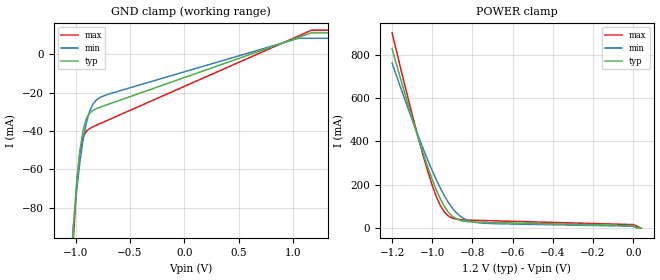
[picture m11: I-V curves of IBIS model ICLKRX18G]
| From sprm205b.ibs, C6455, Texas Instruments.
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|   Model ICLKRX18G
[Model]   ICLKRX18G
Model_type   Input
Polarity   Non-Inverting
C_comp   2.6600pF   1.8070pF   2.7420pF
Vinh =   0.725V
Vinl =   0.475V
[Temperature Range]   25.0000   0.1250k   -40.0000
[Voltage Range]   1.2000V   1.0800V   1.3200V
[GND_clamp]
| voltage   I(typ)   I(min)   I(max)
-1.2V     -536mA     -388.5mA   -700.1mA
-1.05V    -122.6mA   -113.4mA   -139.2mA
-1.02V    -90.24mA   -89.56mA   -96.12mA
-990mV    -66.94mA   -70.92mA   -68.08mA
-960mV    -50.23mA   -56.04mA   -51.12mA
-930mV    -39.33mA   -44.3mA    -43.09mA
-900mV    -33.39mA   -35.52mA   -40.04mA
-870mV    -30.59mA   -29.56mA   -38.7mA
-780mV    -27.67mA   -22.64mA   -36.26mA
1.05V     8.921mA    8.466mA    9.691mA
1.17V     11.32mA    NA         12.7mA
1.32V     11.32mA    8.466mA    12.7mA
[POWER_clamp]
| voltage   I(typ)   I(min)   I(max)
-1.2V     826.7mA    761.5mA    900.4mA
-1.1V     505.9mA    499.6mA    524.1mA
-1.02V    274.4mA    308.1mA    254.4mA
-980mV    176.4mA    223.1mA    146mA
-960mV    135mA      184.7mA    104.5mA
-920mV    73.4mA     118.7mA    55.73mA
-900mV    54.51mA    92.31mA    45.94mA
-860mV    35.69mA    54.58mA    39.13mA
-780mV    27.84mA    26.21mA    36.08mA
0V        11.92mA    8.966mA    16.47mA
20mV      0A         0A         8.235mA
40mV      0A         0A         0A
